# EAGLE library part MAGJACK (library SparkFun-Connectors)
MAGJACK: RJ-45 with LEDs This is a single port, RJ45 ethernet jacks with built in transformer (magnetics), status LEDs, and shielding. Here is the connector we sell at SparkFun: RJ45 Ethernet MagJack-Compatible (PRT-08534) Datasheet It is used on this SparkFun product: SparkFun RJ45 MagJack Breakout (BOB-13021)
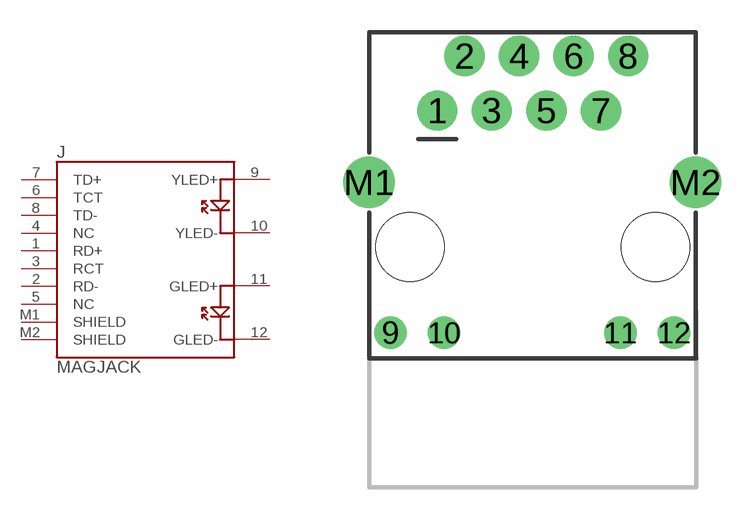
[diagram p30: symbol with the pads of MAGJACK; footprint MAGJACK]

Designator prefix J

## MAGJACK (PROD_ID: CONN-09556; SF_ID: PRT-08534)  [MAGJACK]
1  RD+
2  RD-
3  RCT
4  NC
5  NC
6  TCT
7  TD+
8  TD-
9  YLED+
10  YLED-
11  GLED+
12  GLED-
M1  SHIELD
M2  SHIELD

## Footprint MAGJACK (pad centres in mm)
RJ45 Ethernet MagJack-Compatible tDocu shows where the cable plugs in Specifications: Pin count: 14 Datasheet referenced for footprint Example device(s): MAGJACK
drill 1 pad 1.88: 1 3.175,17.445; 2 4.445,19.985; 3 5.715,17.445; 4 6.985,19.985; 5 8.255,17.445; 6 9.525,19.985; 7 10.795,17.445; 8 12.065,19.985
drill 1 pad 1.27: 9 1,7.1; 10 3.5,7.1; 11 11.7,7.1; 12 14.2,7.1
drill 1.6 pad 2.184: M1 0,14.1; M2 15.2,14.1
hole 3.2 at 1.905,11.095
hole 3.2 at 13.335,11.095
